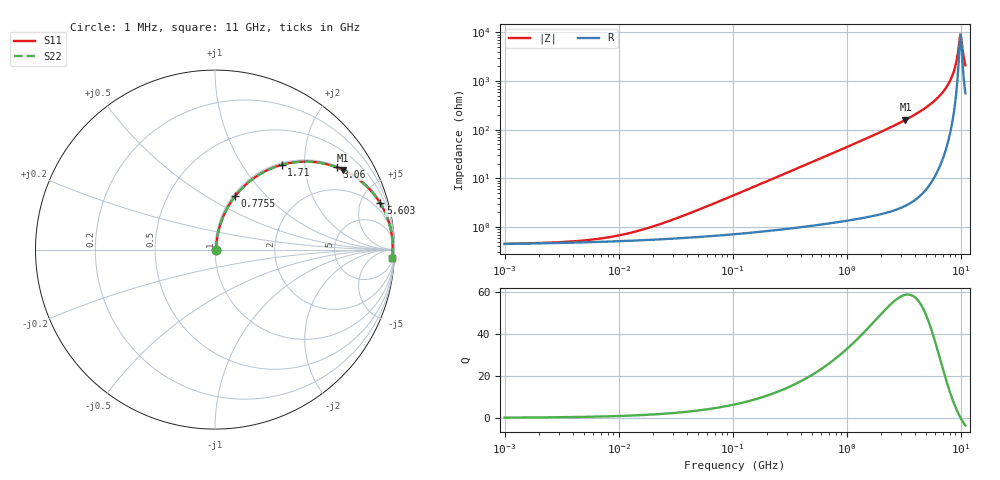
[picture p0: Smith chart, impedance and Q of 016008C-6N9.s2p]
# MHz S MA R 50
!Freq  MagS11  AngS11  MagS21  AngS21  MagS12  AngS12  MagS22  AngS22
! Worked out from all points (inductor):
!   801 points, 1 MHz to 11 GHz, reference 50 ohm
!   read as one part in series: L = 6.9 nH near 41.84 MHz
!   highest Q = 58.5 at 3.281 GHz (marker M1), where L = 7.74 nH
!   self-resonance near 9.907 GHz
!   S11 on the Smith chart (normalised r, x): 1 MHz: 1.01, +0.00; 775.5 MHz: 1.02, +0.68; 1.71 GHz: 1.03, +1.53; 3.06 GHz: 1.05, +2.93; 5.603 GHz: 1.17, +7.10; 11 GHz: 12, -41
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1  0.004486 5.5  0.9955 -0.0  0.9955 -0.0  0.004486 5.5
4.752622  0.005218 23.0  0.9952 -0.1  0.9952 -0.1  0.005218 23.0
10.36096  0.006774 41.0  0.9949 -0.3  0.9949 -0.3  0.006774 41.0
22.3262  0.01109 59.6  0.9944 -0.6  0.9944 -0.6  0.01109 59.6
104.8809  0.04566 78.5  0.9919 -2.6  0.9919 -2.6  0.04566 78.5
248.042  0.1064 79.3  0.9858 -6.1  0.9858 -6.1  0.1064 79.3
498.4592  0.2099 75.1  0.9675 -12.1  0.9675 -12.1  0.2099 75.1
775.5249  0.3172 69.4  0.937 -18.5  0.937 -18.5  0.3172 69.4
1165.217  0.4509 61.6  0.8801 -26.8  0.8801 -26.8  0.4509 61.6
1710.465  0.6009 51.8  0.7862 -36.9  0.7862 -36.9  0.6009 51.8
2341.592  0.7253 42.4  0.6749 -46.5  0.6749 -46.5  0.7253 42.4
3059.857  0.8194 34.0  0.5593 -55.0  0.5593 -55.0  0.8194 34.0
3281.041  0.8409 31.8  0.527 -57.2  0.527 -57.2  0.8409 31.8
5602.627  0.9565 15.6  0.2693 -73.0  0.2693 -73.0  0.9565 15.6
6988.352  0.9793 9.5  0.1644 -78.1  0.1644 -78.1  0.9793 9.5
8129.193  0.9875 5.4  0.0941 -79.7  0.0941 -79.7  0.9875 5.4
8921.982  0.9896 2.9  0.05164 -76.9  0.05164 -76.9  0.9896 2.9
9566.912  0.9898 1.1  0.02131 -60.9  0.02131 -60.9  0.9898 1.1
9906.655  0.9895 0.2  0.01091 -15.0  0.01091 -15.0  0.9895 0.2
10258.46  0.9888 -0.8  0.01717 49.0  0.01717 49.0  0.9888 -0.8
10747.05  0.9875 -2.0  0.03634 68.9  0.03634 68.9  0.9875 -2.0
11000  0.9866 -2.6  0.04661 72.0  0.04661 72.0  0.9866 -2.6
